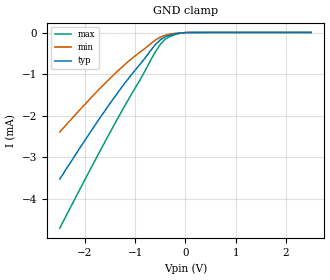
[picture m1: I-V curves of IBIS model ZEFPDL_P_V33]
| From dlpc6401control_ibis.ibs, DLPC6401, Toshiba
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|   Model ZEFPDL_P_V33
[Model]   ZEFPDL_P_V33
Model_type   Input
Vinh = 1.25
Vinl = 1.15
Polarity   Non-Inverting
C_comp   1.0e-12   1.0e-12   1.0e-12
[Voltage Range]   3.300V   3.000V   3.600V
[Temperature Range]   25.000   125.000   -40
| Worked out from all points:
|   GND clamp passes 1 mA (typ) near -1.06 V on its own axis
[GND_clamp]
| voltage   I(typ)   I(min)   I(max)
-2.5V     -3.53mA    -2.394mA   -4.711mA
-1.8V     -2.232mA   -1.469mA   -3.082mA
-1.3V     -1.37mA    -872.9uA   -1.964mA
-900mV    -757uA     -464.6uA   -1.131mA
-600mV    -290.7uA   -181.2uA   -465.9uA
-500mV    -171.7uA   -107.8uA   -283uA
-400mV    -97.96uA   -61.48uA   -155uA
-200mV    -29.78uA   -17.87uA   -46.34uA
0V        -35.48pA   -30.26pA   -53.49pA
2.5V      4.002uA    3.056uA    5.487uA
[POWER_clamp]
| voltage   I(typ)   I(min)   I(max)
-2.5V     0A         NA         NA
0V        0A         NA         NA
